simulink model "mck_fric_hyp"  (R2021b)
settings: Solver=VariableStepAuto  StartTime=0.0  StopTime=20  RelTol=1e-3
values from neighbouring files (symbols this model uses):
  C = 1    [mck_fric.m]
  K = 10    [mck_fric.m]
  M = 1    [mck_fric.m]
undefined symbols (not defined in the file or in its folder): BLDC, dynamics
libraries: fl_lib x9, nesl_utility x4

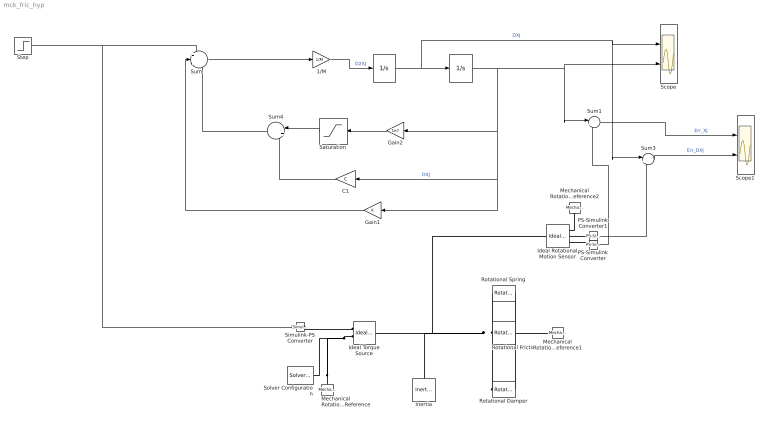
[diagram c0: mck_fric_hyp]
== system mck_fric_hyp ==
  " " : Integrator
  "  " : Integrator  UpperSaturationLimit=dynamics.ThUmax/dynamics.tau  LowerSaturationLimit=dynamics.ThUmin/dynamics.tau
  1/M : Gain  Gain=1/M
  C1 : Gain  Gain=C
  Gain1 : Gain  Gain=K
  Gain2 : Gain  Gain=1e7
  Ideal Rotational Motion Sensor : fl_lib/Mechanical/Mechanical Sensors/Ideal Rotational Motion Sensor  wrap_angle=simscape.enum.onoff.off  offset=0 rad
  Ideal Torque Source : fl_lib/Mechanical/Mechanical Sources/Ideal Torque Source
  Inertia : fl_lib/Mechanical/Rotational Elements/Inertia  inertia=M kg*m^2  num_ports=foundation.enum.numPorts2.one  w_specify=off  w_priority=High  w=0 rad/s  w_nominal_specify=off  w_nominal_unit=rad/s  w_nominal_value=1  t_specify=off  t_priority=None  t=0 N*m  t_nominal_specify=off  t_nominal_unit=N*m  t_nominal_value=1
  Mechanical Rotational Reference : fl_lib/Mechanical/Rotational Elements/Mechanical Rotational Reference
  Mechanical Rotational Reference1 : fl_lib/Mechanical/Rotational Elements/Mechanical Rotational Reference
  Mechanical Rotational Reference2 : fl_lib/Mechanical/Rotational Elements/Mechanical Rotational Reference
  PS-Simulink Converter : nesl_utility/PS-Simulink Converter  PhysicalDomain=network_engine_domain  SubClassName=ps_output  LeftPortType=input  RightPortType=output  PseudoPeriodic=off  Frequencies=[]  Unit=inherit  AffineConversion=off
  PS-Simulink Converter1 : nesl_utility/PS-Simulink Converter  PhysicalDomain=network_engine_domain  SubClassName=ps_output  LeftPortType=input  RightPortType=output  PseudoPeriodic=off  Frequencies=[]  Unit=inherit  AffineConversion=off
  Rotational Damper : fl_lib/Mechanical/Rotational Elements/Rotational Damper  D=C N*m/(rad/s)  w_specify=off  w_priority=None  w=0 rad/s  w_nominal_specify=off  w_nominal_unit=rad/s  w_nominal_value=1  t_specify=off  t_priority=None  t=0 N*m  t_nominal_specify=off  t_nominal_unit=N*m  t_nominal_value=1
  Rotational Friction : fl_lib/Mechanical/Rotational Elements/Rotational Friction  brkwy_trq=dynamics.friction.FDTm*BLDC.TMM N*m  brkwy_vel=0.00001201 rad/s  Col_trq=dynamics.friction.FDTm*BLDC.TMM N*m  visc_coef=0 N*m/(rad/s)  w_specify=off  w_priority=None  w=0 rad/s  w_nominal_specify=off  w_nominal_unit=rad/s  w_nominal_value=1  t_specify=off  t_priority=None  t=0 N*m  t_nominal_specify=off  t_nominal_unit=N*m  t_nominal_value=1
  Rotational Spring : fl_lib/Mechanical/Rotational Elements/Rotational Spring  spr_rate=K N*m/rad  w_specify=off  w_priority=None  w=0 rad/s  w_nominal_specify=off  w_nominal_unit=rad/s  w_nominal_value=1  t_specify=off  t_priority=None  t=0 N*m  t_nominal_specify=off  t_nominal_unit=N*m  t_nominal_value=1  phi_specify=off  phi_priority=High  phi=0 rad  phi_nominal_specify=off  phi_nominal_unit=rad  phi_nominal_value=1
  Saturation : Saturate  UpperLimit=dynamics.friction.FDTm*BLDC.TMM  LowerLimit=-dynamics.friction.FDTm*BLDC.TMM
  Scope : Scope  NumInputPorts=2
  Scope1 : Scope  NumInputPorts=2
  Simulink-PS Converter : nesl_utility/Simulink-PS Converter  PhysicalDomain=network_engine_domain  SubClassName=ps_input  LeftPortType=input  RightPortType=output  PseudoPeriodic=off  Frequencies=[]  NoiseDistribution=none  NoiseParameters=[]  Unit=1  AffineConversion=off  FilteringAndDerivatives=provide  SimscapeFilterOrder=1  InputFilterTimeConstant=0.001  UdotUserProvided=0
  Solver Configuration : nesl_utility/Solver Configuration  PhysicalDomain=network_engine_domain  SubClassName=solver  LeftPortType=input  RightPortType=generic  Tones=[]  Harmonics=[]  SimulateNoise=off  Profile=off  UseLocalSampling=off  EnableSwitchedLinearOptims=on  FrequencyDomain=off  UseCCode=off  RelTol=0.001  AbsTol=1e-06  MinStep=1e-09  ToWorkspace=off  RevertToSquareIcSolve=off  NumHomotopyIterations=100  PhasorMode=off  PhasorModeNumHarmonics=1  DoDC=off  ResidualTolerance=1e-09  UseLocalSolver=off  LocalSolverChoice=NE_BACKWARD_EULER_ADVANCER  LocalSolverSampleTime=0.001  DoFixedCost=off  MaxNonlinIter=3  MaxModeIter=2  ComputeImpulses=off  ImpulseIterations=2  LinearAlgebra=auto  EquationFormulation=NE_TIME_EF  DelaysMemoryBudget=1024  AutomaticFiltering=on  FilteringTimeConstant=0.001  PartitionStorageMethod=AS_NEEDED  PartitionMemoryBudget=1024  PartitionMethod=ROBUST
  Step : Step  Time=10  Before=0.5  After=-0.5  SampleTime=0
  Sum : Sum  Inputs=+--
  Sum1 : Sum  Inputs=|+-
  Sum3 : Sum  Inputs=|+-
  Sum4 : Sum  Inputs=|++
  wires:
  Sum/1 -> 1/M/1
  1/M/1 -> " "/1  "D2XJ"
  " "/1 -> Sum3/1, Scope/1, "  "/1  "DXJ"
  Gain1/1 -> Sum/2
  PS-Simulink Converter/1 -> Sum1/2
  Sum1/1 -> Scope1/1  "Err_XJ"
  PS-Simulink Converter1/1 -> Sum3/2
  Sum3/1 -> Scope1/2  "Err_DXJ"
  Step/1 -> Simulink-PS Converter/1, Sum/1
  Saturation/1 -> Sum4/1
  Sum4/1 -> Sum/3
  C1/1 -> Sum4/2
  Gain2/1 -> Saturation/1
  "  "/1 -> Sum1/1, Scope/2, C1/1, Gain1/1, Gain2/1  "DXJ"
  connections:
  Ideal Torque Source/RConn2 -- Mechanical Rotational Reference/LConn1 -- Solver Configuration/RConn1
  Simulink-PS Converter/RConn1 -- Ideal Torque Source/RConn1
  Rotational Damper/LConn1 -- Ideal Rotational Motion Sensor/LConn1 -- Inertia/LConn1 -- Ideal Torque Source/LConn1 -- Rotational Spring/LConn1 -- Rotational Friction/LConn1
  Rotational Spring/RConn1 -- Mechanical Rotational Reference1/LConn1 -- Rotational Damper/RConn1 -- Rotational Friction/RConn1
  PS-Simulink Converter1/LConn1 -- Ideal Rotational Motion Sensor/RConn2
  Mechanical Rotational Reference2/LConn1 -- Ideal Rotational Motion Sensor/RConn1
  PS-Simulink Converter/LConn1 -- Ideal Rotational Motion Sensor/RConn3
